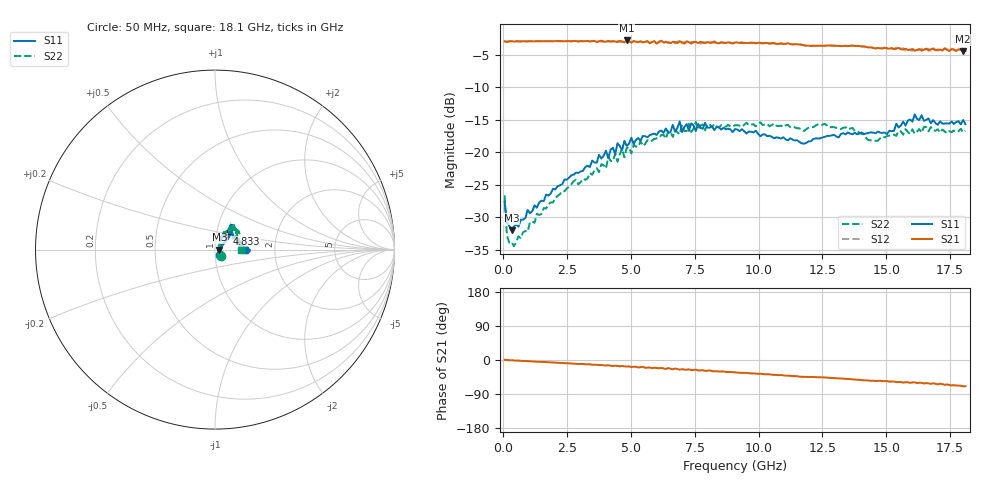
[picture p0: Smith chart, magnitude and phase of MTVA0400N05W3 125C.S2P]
! Network Analyzer HP8720D.06.14 Serial No. US36140669
!  8 Jul 2005  06:48:01
! Frequency  S11  S21  S12  S22
# HZ  S  DB R 50
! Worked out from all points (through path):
!   201 points, 50 MHz to 18.1 GHz, reference 50 ohm
!   highest |S21| = -2.78 dB at 4.833 GHz (marker M1); lowest = -4.4 dB at 18.01 GHz (marker M2)
!   group delay of S21, straight-line fit = 10.6 ps
!   lowest |S11| = -32.0 dB at 320.8 MHz (marker M3), VSWR 1.05, Z = 52.6 - j0.0701 ohm
!   |S11| at or under -10 dB: start of sweep to end of sweep
!   |S22| runs from -34.5 to -15.3 dB; largest |S21 - S12| = 0.032
!   S11 on the Smith chart (normalised r, x): 50 MHz: 1.06, -0.06; 4.833 GHz: 1.13, +0.20; 18.1 GHz: 1.39, -0.01
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5e7  -27.68 -44.7  -2.91 0.6  -2.94 0.7  -26.64 -45.1
1.4025e8  -30.81 -25.4  -2.99 -0.2  -2.98 -0.2  -32.83 -30.5
3.2075e8  -32.04 -1.5  -2.89 -0.6  -2.92 -0.6  -33.79 -2.0
3.1185e9  -22.87 39.8  -2.89 -10.3  -2.93 -10.7  -24.09 58.7
4.021e9  -19.76 44.7  -2.94 -14.6  -2.92 -13.7  -22.50 58.0
4.11125e9  -20.93 45.1  -2.87 -13.7  -2.96 -14.7  -20.68 58.4
4.47225e9  -18.61 42.8  -3.03 -15.6  -2.85 -15.2  -21.48 63.4
4.83325e9  -19.03 52.2  -2.78 -17.1  -2.97 -17.4  -19.35 53.8
6.09675e9  -16.80 49.9  -3.04 -21.9  -2.93 -21.8  -17.81 55.3
6.7285e9  -16.85 55.5  -3.01 -22.4  -3.26 -22.9  -16.54 50.0
6.909e9  -15.26 53.5  -2.89 -25.6  -2.93 -24.0  -17.25 50.4
6.99925e9  -16.89 53.0  -3.06 -24.2  -3.25 -25.7  -15.77 51.2
7.36025e9  -15.56 48.5  -3.27 -26.4  -2.97 -25.9  -16.86 54.2
7.54075e9  -16.72 50.6  -3.03 -25.4  -2.96 -27.9  -15.33 52.5
7.90175e9  -15.48 53.3  -3.19 -28.6  -3.04 -27.4  -16.61 47.9
9.075e9  -16.43 51.2  -3.11 -32.5  -3.08 -32.7  -15.85 40.9
1.21435e10  -17.96 30.0  -3.62 -44.7  -3.55 -45.0  -16.15 43.2
1.512175e10  -16.69 3.7  -4.05 -57.0  -3.88 -57.0  -17.45 27.3
1.61145e10  -14.19 -1.2  -4.36 -59.0  -4.01 -60.0  -17.15 19.2
1.7017e10  -15.78 -4.5  -4.19 -64.4  -4.36 -65.4  -16.47 8.9
1.800975e10  -15.03 -3.3  -4.44 -69.5  -4.25 -70.7  -16.95 5.6
1.81e10  -15.68 -1.3  -4.41 -69.1  -4.50 -69.0  -16.70 -0.6
